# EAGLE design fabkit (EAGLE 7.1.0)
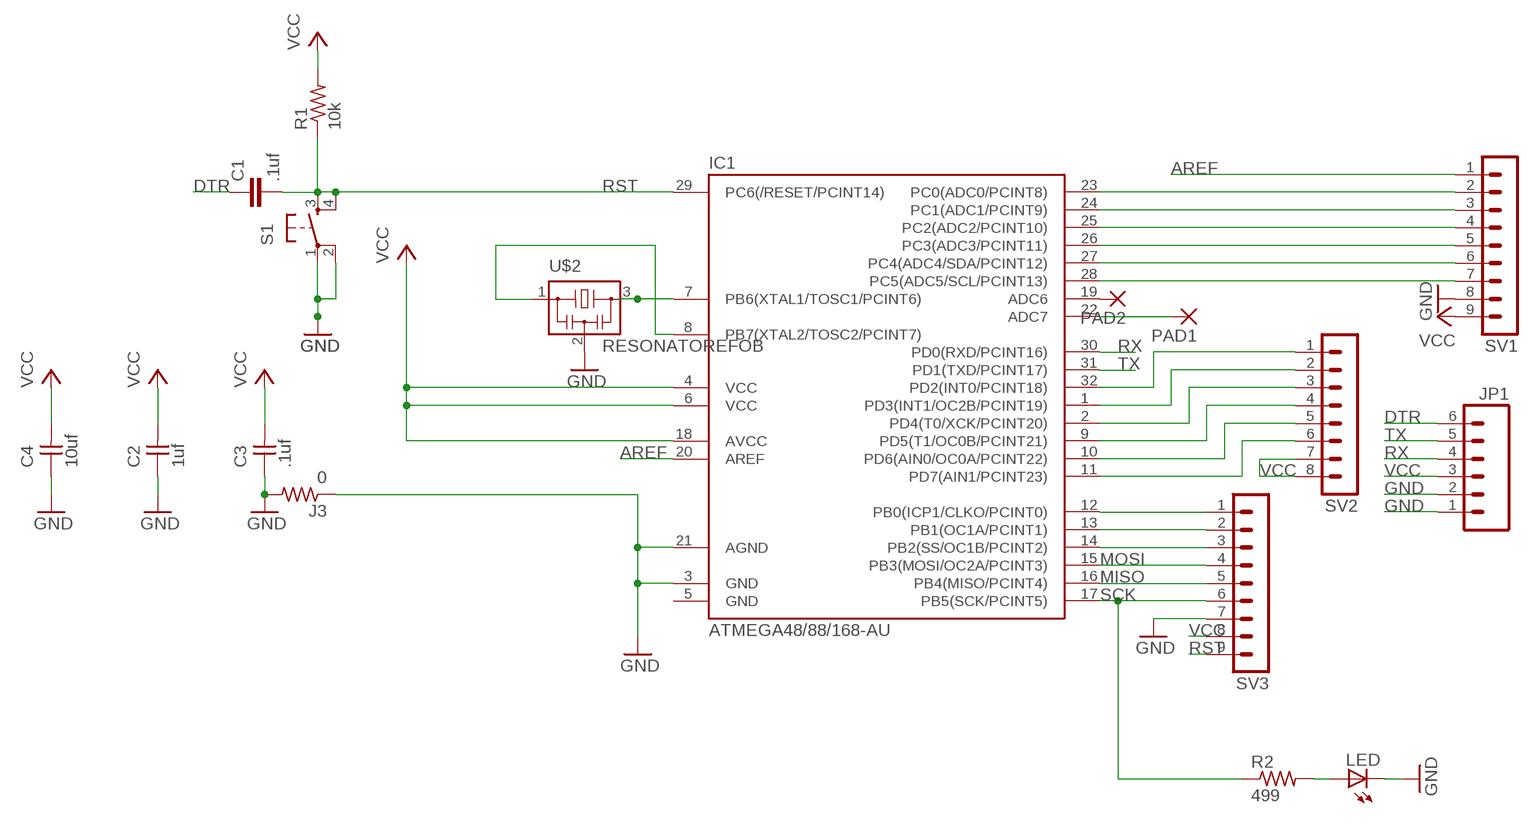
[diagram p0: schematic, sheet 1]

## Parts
C1  .1uf  C-EUC1206  [C1206]
C2  1uf  UNPOLARIZED_CAPACITOR1206  [1206]
C3  .1uf  UNPOLARIZED_CAPACITOR1206  [1206]
C4  10uf  UNPOLARIZED_CAPACITOR1206  [1206]
IC1  ATMEGA48/88/168-AU  [TQFP32-08]
J3  0  RESISTOR1206  [1206]
JP1  M06SMD  [1X06-SMD]
LED  LED1206  [1206]
PAD1  1,6/0,8  [1,6/0,8]
PAD2  1,6/0,8  [1,6/0,8]
R1  10k  RESISTOR1206  [1206]
R2  499  RESISTOR1206  [1206]
S1  6MM_SWITCH6MM_SWITCH  [6MM_SWITCH]
SV1  MA09-1  [MA09-1]
SV2  MA08-1  [MA08-1]
SV3  MA09-1  [MA09-1]
U$2  RESONATOREFOB  [EFOBM]

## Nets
AREF: IC1.20(AREF) SV1.1
DTR: C1.1 JP1.6
GND: C2.1 C3.1 C4.1 IC1.3(GND) IC1.21(AGND) J3.1 J3.2 JP1.1 JP1.2 LED.2(C) S1.1(P) S1.2(P1) SV1.8 SV3.7 U$2.2
MISO: IC1.16(PB4(MISO/PCINT4)) SV3.5
MOSI: IC1.15(PB3(MOSI/OC2A/PCINT3)) SV3.4
N$1: IC1.8(PB7(XTAL2/TOSC2/PCINT7)) U$2.1
N$2: IC1.12(PB0(ICP1/CLKO/PCINT0)) SV3.1
N$3: IC1.23(PC0(ADC0/PCINT8)) SV1.2
N$4: IC1.24(PC1(ADC1/PCINT9)) SV1.3
N$5: IC1.25(PC2(ADC2/PCINT10)) SV1.4
N$6: IC1.26(PC3(ADC3/PCINT11)) SV1.5
N$7: IC1.27(PC4(ADC4/SDA/PCINT12)) SV1.6
N$8: IC1.28(PC5(ADC5/SCL/PCINT13)) SV1.7
N$9: IC1.7(PB6(XTAL1/TOSC1/PCINT6)) U$2.3
N$10: IC1.32(PD2(INT0/PCINT18)) SV2.1
N$11: IC1.1(PD3(INT1/OC2B/PCINT19)) SV2.2
N$12: IC1.2(PD4(T0/XCK/PCINT20)) SV2.3
N$13: IC1.9(PD5(T1/OC0B/PCINT21)) SV2.4
N$14: IC1.10(PD6(AIN0/OC0A/PCINT22)) SV2.5
N$15: IC1.11(PD7(AIN1/PCINT23)) SV2.6
N$16: IC1.22(ADC7) PAD1.1(P)
N$17: IC1.13(PB1(OC1A/PCINT1)) SV3.2
N$18: IC1.14(PB2(SS/OC1B/PCINT2)) SV3.3
N$19: IC1.19(ADC6) PAD2.1(P)
N$23: LED.1(A) R2.2
RST: C1.2 IC1.29(PC6(/RESET/PCINT14)) R1.1 S1.3(S) S1.4(S1) SV3.9
RX: IC1.30(PD0(RXD/PCINT16)) JP1.4
SCK: IC1.17(PB5(SCK/PCINT5)) R2.1 SV3.6
TX: IC1.31(PD1(TXD/PCINT17)) JP1.5
VCC: C2.2 C3.2 C4.2 IC1.4(VCC) IC1.6(VCC) IC1.18(AVCC) JP1.3 R1.2 SV1.9 SV2.7 SV2.8 SV3.8

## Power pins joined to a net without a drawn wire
GND: IC1.5(GND)

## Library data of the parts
C1 = rcl:C-EU: CAPACITOR, European symbol
C2-C4 = ng:UNPOLARIZED_CAPACITOR: unpolarized_capacitor
IC1 = atmega8:ATMEGA48/88/168
J3 R1 R2 = ng:RESISTOR
JP1 = SparkFun:M06: Header 6 Standard 6-pin 0.1" header. Use with straight break away headers (SKU : PRT-00116), right angle break away headers (PRT-00553), swiss pins (PRT-00743), machine pins (PRT-00117), and female headers (PRT-00115). Molex polarized connector foot print use with SKU : PRT-08094 with associated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
LED = ng:LED
PAD1 PAD2 = wirepad:1,6/0,8: THROUGH-HOLE PAD
S1 = ng:6MM_SWITCH: OMRON SWITCH
SV1 SV3 = con-lstb:MA09-1: PIN HEADER; OC_FARNELL: unknown; OC_NEWARK: unknown
SV2 = con-lstb:MA08-1: PIN HEADER
U$2 = fab:RESONATOR

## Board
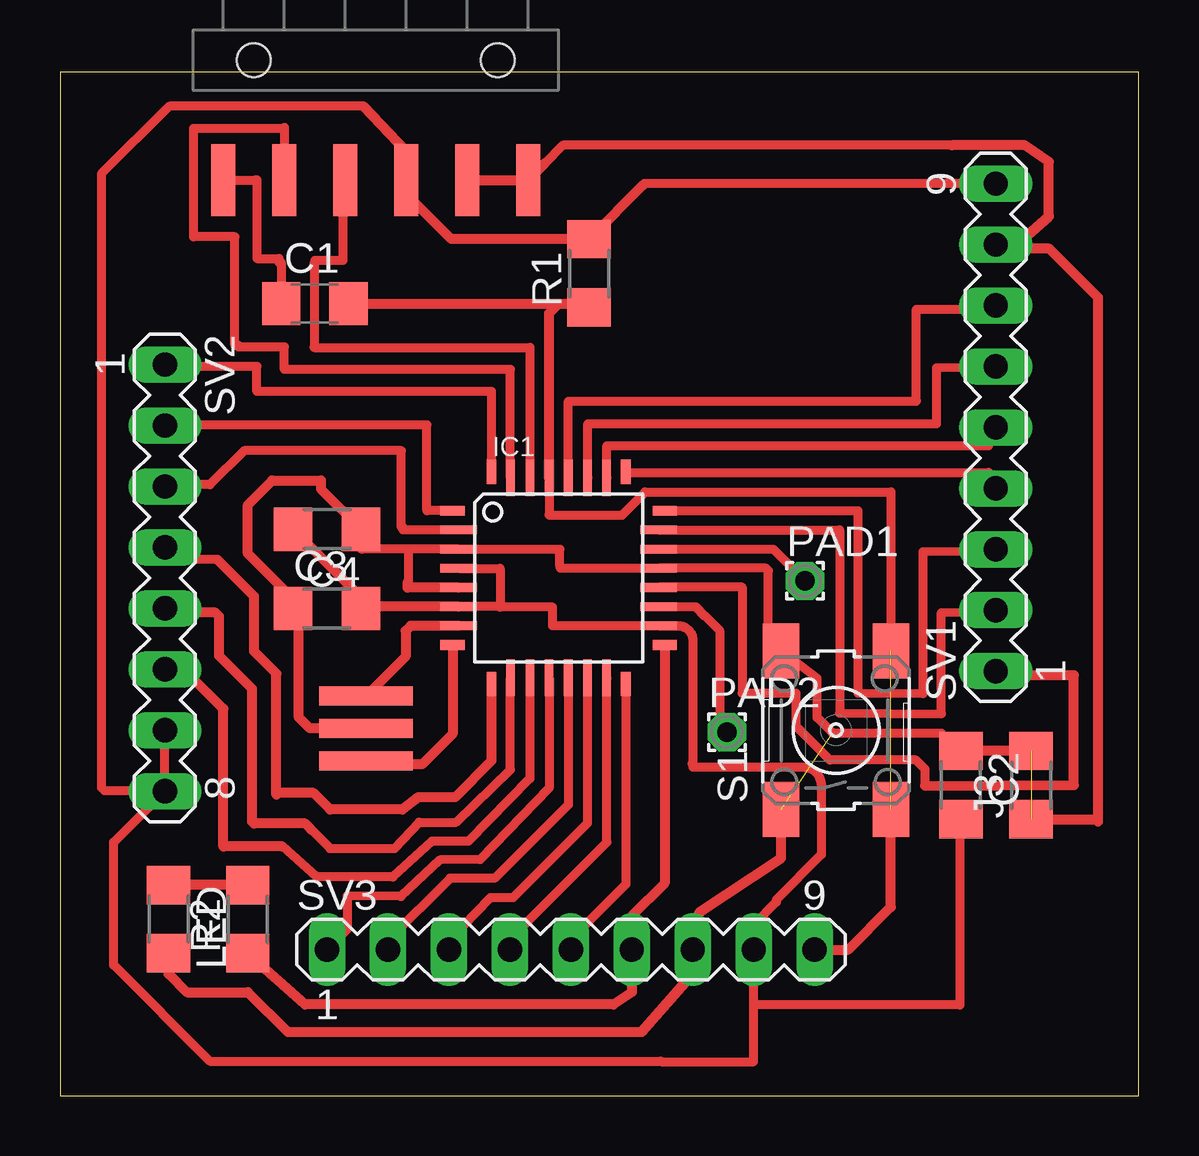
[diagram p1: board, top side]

Size 44.96 x 42.66 mm. Coordinates in mm from the lower left corner, seen from the top.
Outline: 0,0 44.96,0 44.96,42.66 0,42.66 0,0
Copper layers (1*16): Top 0.035mm / dielectric 1.5mm / Bottom 0.035mm
Design rules "default *": minimum track width 14mil, minimum drill 24mil, track to track 15mil, track to pad 15mil, pad to pad 15mil, via to via 15mil, smd to smd 15mil, copper to edge 40mil, drill to drill 8mil, minimum pad ring 10mil, minimum via ring 8mil, stop-mask expansion 4mil, vias tented up to drill 0mil, thermal gap 10mil

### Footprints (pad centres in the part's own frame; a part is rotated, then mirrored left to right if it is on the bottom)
C1206 = smd 1.6 x 1.8: 1 -1.4,0; 2 1.4,0
1206 = smd 1.6 x 1.803: 1 -1.422,0; 2 1.422,0
TQFP32-08 = smd 1.016 x 0.406: 1 -4.42,2.8; 8 -4.42,-2.8; 17 4.42,-2.8; 24 4.42,2.8 | smd 1.524 x 0.356: 2 -4.166,2; 3 -4.166,1.2; 4 -4.166,0.4; 5 -4.166,-0.4; 6 -4.166,-1.2; 7 -4.166,-2; 18 4.166,-2; 19 4.166,-1.2; 20 4.166,-0.4; 21 4.166,0.4; 22 4.166,1.2; 23 4.166,2 | smd 0.406 x 1.016: 9 -2.8,-4.42; 16 2.8,-4.42; 25 2.8,4.42; 32 -2.8,4.42 | smd 0.356 x 1.524: 10 -2,-4.166; 11 -1.2,-4.166; 12 -0.4,-4.166; 13 0.4,-4.166; 14 1.2,-4.166; 15 2,-4.166; 26 2,4.166; 27 1.2,4.166; 28 0.4,4.166; 29 -0.4,4.166; 30 -1.2,4.166; 31 -2,4.166
1X06-SMD = smd 1 x 3: 1 -6.35,5; 2 -3.81,5; 3 -1.27,5; 4 1.27,5; 5 3.81,5; 6 6.35,5 | hole 1.4: -5.08,0; 5.08,0
1,6/0,8 = drill 0.813 pad 1.6 octagon: 1 0,0
6MM_SWITCH = smd 2.286 x 1.524: 1 -3.302,2.286; 2 3.302,2.286; 3 -3.302,-2.286; 4 3.302,-2.286
MA09-1 = drill 1.016 long: 1 -10.16,0; 2 -7.62,0; 3 -5.08,0; 4 -2.54,0; 5 0,0; 6 2.54,0; 7 5.08,0; 8 7.62,0; 9 10.16,0
MA08-1 = drill 1.016 long: 1 -8.89,0; 2 -6.35,0; 3 -3.81,0; 4 -1.27,0; 5 1.27,0; 6 3.81,0; 7 6.35,0; 8 8.89,0
EFOBM = smd 0.8 x 3.9: 1 -1.35,0; 2 0,0; 3 1.35,0

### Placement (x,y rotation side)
C1  10.62,33.02 0 top
C2  37.54,12.95 270 top
C3  11.13,20.32 0 top
C4  11.13,23.62 180 top
IC1  20.78,21.59 0 top
J3  40.46,12.95 90 top
JP1  13.16,43.18 180 top
LED  4.52,7.37 270 top
PAD1  31.04,21.46 0 top
PAD2  27.79,15.16 0 top
R1  22.05,34.29 90 top
R2  7.82,7.37 90 top
S1  32.33,15.24 90 top
SV1  38.99,27.86 90 top
SV2  4.37,21.59 270 top
SV3  21.29,6.1 0 top
U$2  12.75,15.32 90 top

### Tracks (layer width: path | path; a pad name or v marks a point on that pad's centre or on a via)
AREF
  Top 0.381: 36.04,12.93 36.04,13.61 35.66,14 32.08,14 30.66,15.42 30.66,16.79 28.42,16.79 28.42,21.21 24.94,21.21 IC1.20
  Top 0.406: 38.81,17.65 SV1.1 38.81,17.53 42.24,17.53 42.24,12.95 36.04,12.93
DTR
  Top 0.381: JP1.6 8.15,38.18 8.2,38.18 8.2,34.9 9.12,34.9 9.12,34.75 9.22,34.75 C1.1
GND  (2 unrouted)
  Top 0.381: 14.53,22.79 IC1.3 20.83,22.78 20.83,22.07 20.85,22.07 20.85,21.99 IC1.21 29.41,22 29.52,21.89 29.52,18.67 29.64,18.54 S1.2 31.55,17.4 31.55,15.77 32.18,15.14 32.18,15.11 36.73,15.11 C2.1 | 14.53,22.79 12.57,22.79 12.57,22.81 12.55,22.81 C4.1 | 14.48,21.19 14.48,21.44 14.53,21.44 14.53,22.79 | 37.16,39.62 20.95,39.62 20.19,38.86
  Top 0.406: JP1.2 JP1.1 20.19,38.86 | C4.1 10.87,25.3 10.87,25.65 8.84,25.65 7.82,24.64 7.82,22.61 9.7,20.73 C3.1 9.96,20.07 9.96,15.77 10.41,15.32 U$2.2 | S1.1 30.05,9.91 26.62,7.62 26.62,6.35 SV3.7 26.37,5.08 24.23,2.67 9.5,2.67 7.82,4.32 5.28,4.32 4.52,5.08 LED.2 | 37.16,39.62 40.21,39.62 41.2,38.94 41.2,36.65 39.83,35.43 SV1.8 38.81,35.31 41.22,35.31 43.26,33.27 43.26,11.43 43.15,11.53 J3.1 | J3.2 C2.1 | IC1.5 14.48,21.19
MISO
  Top 0.381: IC1.16 23.58,8.82 21.29,6.53 SV3.5
MOSI
  Top 0.381: SV3.4 18.75,6.53 22.78,10.57 IC1.15
N$1
  Top 0.406: IC1.8 16.36,15.09 15.09,13.82 12.9,13.82 U$2.1
N$2
  Top 0.381: IC1.12 20.38,12.83 17.5,9.86 15.82,9.83 14.2,8.31 11.96,8.33 11.96,6.93 SV3.1
N$3
  Top 0.381: IC1.23 32.49,23.59 32.49,15.95 36.73,15.93 36.73,20.14 38.68,20.17 SV1.2
N$4
  Top 0.381: IC1.24 33.25,24.39 33.25,16.79 35.97,16.76 35.97,22.68 38.68,22.71 SV1.3
N$5
  Top 0.381: IC1.25 23.55,26.01 23.55,25.98 38.68,25.98 SV1.4
N$6
  Top 0.381: IC1.26 22.78,27.1 38.68,27.1 SV1.5
N$7
  Top 0.381: IC1.27 22,25.76 22,28.02 36.53,28.02 36.53,30.35 SV1.6
N$8
  Top 0.381: IC1.28 21.18,28.96 35.66,28.96 35.66,28.98 35.69,28.98 35.69,32.79 38.68,32.79 SV1.7
N$9
  Top 0.406: IC1.7 14.61,19.59 14.4,19.38 14.4,18.32 U$2.3
N$10
  Top 0.381: IC1.32 17.98,29.36 8.2,29.36 8.2,30.4 4.45,30.4 SV2.1
N$11
  Top 0.381: IC1.1 15.29,24.39 15.29,27.96 4.39,27.96 SV2.2
N$12
  Top 0.381: IC1.2 14.3,23.59 14.3,23.7 14.22,23.7 14.22,26.9 7.67,26.9 6.25,25.48 4.45,25.48 SV2.3
N$13
  Top 0.381: 6.55,22.35 4.88,22.35 SV2.4
  Top 0.406: IC1.9 17.98,13.96 16.46,12.45 14.94,12.45 14.28,11.94 11.25,11.94 10.57,12.62 9.09,12.62 9.02,12.55 9.02,17.6 8.08,18.54 8.08,20.83 6.55,22.35
N$14
  Top 0.381: 10.47,11.1 11.25,10.31 13.94,10.31 14.96,11.41 16.51,11.41 18.77,13.59 IC1.10
  Top 0.406: 10.47,11.1 10.21,11.35 8.08,11.35 8,11.43 8,16.97 6.63,18.34 6.63,19.99 6.48,20.14 4.37,20.14 SV2.5
N$15
  Top 0.381: IC1.11 19.58,13.23 17.02,10.62 15.49,10.62 13.87,9.12 10.69,9.12 9.27,10.39 | 5.31,17.78 SV2.6
  Top 0.406: 9.27,10.39 6.81,10.39 6.81,16.13 5.16,17.78 SV2.6
N$16
  Top 0.381: IC1.22 29.71,22.79 PAD1.1
N$17
  Top 0.381: IC1.13 21.18,12.14 18.11,9.07 16.26,9.07 13.67,6.48 SV3.2
N$18
  Top 0.381: IC1.14 21.98,11.36 18.87,8.25 17.93,8.25 16.21,6.45 SV3.3
N$19
  Top 0.381: IC1.19 26.47,20.39 26.87,19.99 26.9,19.99 27.48,19.41 27.48,15.47 PAD2.1
N$23
  Top 0.406: R2.2 LED.1
RST  (1 unrouted)
  Top 0.381: IC1.29 20.38,24.23 20.4,24.21 23.42,24.21 24.38,25.17 34.62,25.17 S1.4 34.52,18.64 34.52,19.43
  Top 0.406: C1.2 20.78,33.02 | 20.78,33.02 21.9,33.02 R1.1 | IC1.29 20.38,32.62 20.78,33.02 | SV3.9 32.84,6.1 34.62,7.87 S1.3
RX
  Top 0.381: JP1.4 11.79,38.18 11.79,34.82 10.62,34.82 10.62,34.7 10.59,34.7 10.59,31.19 19.58,31.19 | 19.58,31.19 | 19.58,31.19 IC1.30
SCK
  Top 0.406: R2.1 10.21,3.81 23.06,3.81 23.83,4.32 SV3.6 23.83,7.49 25.2,8.87 IC1.17
TX
  Top 0.381: IC1.31 18.77,30.28 9.35,30.28 9.35,31.22 7.44,31.22 7.44,31.29 7.29,31.29 7.29,35.81 5.56,35.81 5.56,40.34 9.35,40.34 | 9.35,40.34 9.35,40.36 | 9.35,40.34 JP1.5
VCC
  Top 0.381: IC1.4 18.34,21.99 18.34,20.4 | 18.34,20.4 IC1.6 | 18.34,20.4 18.34,20.37 20.52,20.37 20.52,19.59 IC1.18 25.72,19.59 arc-90 26.37,19.05 26.37,13.92 26.34,13.84 26.37,13.84 26.37,13.69 30.99,13.69 arc-90 31.72,12.95 31.72,10.06 29.85,8.18 29.85,8.08 28.91,7.14 SV3.8 28.91,3.79 | C2.2 37.49,11.53 37.49,3.79 28.91,3.79 | SV1.9 24.36,38.02 24.31,37.97 | 28.91,3.79 28.91,1.42 25.04,1.42 25.02,1.45 6.25,1.45 2.24,5.46 2.24,10.57 SV2.8 4.34,12.73 | 12.65,41.25 4.55,41.25 1.73,38.43 1.73,12.85 1.85,12.73 4.34,12.73 | 4.34,12.73 4.37,12.75 SV2.7
  Top 0.406: IC1.6 12.33,20.39 12.14,20.57 12.29,20.57 C3.2 12.55,20.78 C4.2 | 12.65,41.25 14.43,39.37 JP1.3 14.43,37.59 16.31,35.71 R1.2 24.31,37.97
